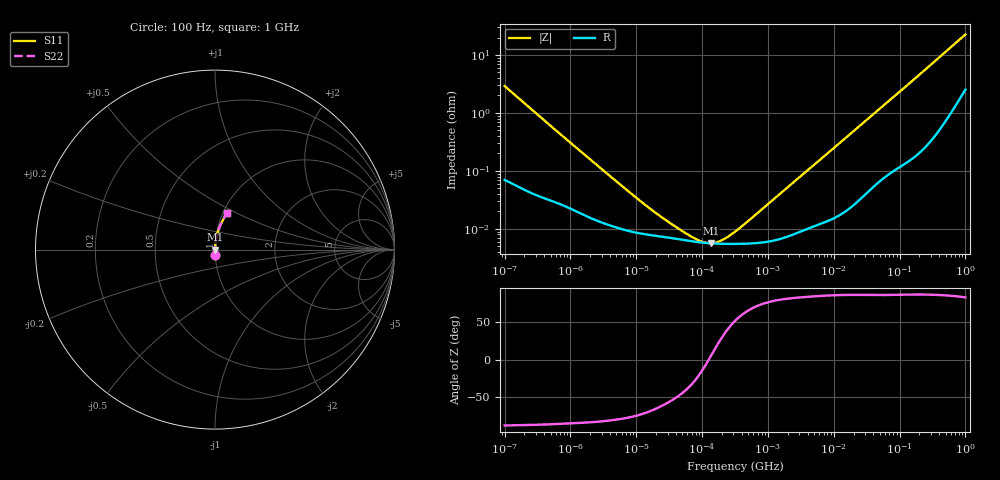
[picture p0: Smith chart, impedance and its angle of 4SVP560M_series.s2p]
!  *** S-Parameter ***
!  Copyright (C) Panasonic Industry Corporation
!  Conductive Polymer Aluminum Soild Capacitor (OS-CON)
!  Parts No. 4SVP560M
!  Connection Mode : Series
!  1  o---||---o  2
!  GND o--------o GND
!  Conditions : Temperature = 20 degC  DC Bias = 0 V
! Frequency Range : 100Hz  -  1GHz  [ 401 Steps ]
# Hz S RI R 50
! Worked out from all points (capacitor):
!   401 points, 100 Hz to 1 GHz, reference 50 ohm
!   read as one part in series: C = 545 uF near 108.4 Hz
!   lowest |Z| = 5.66 mohm at 135.7 kHz (marker M1)
!   series resonance near 126.6 kHz, so ESL is about 2.9 nH
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100  0.00154 -0.029  0.9985 0.029  0.9985 0.029  0.00154 -0.029
108.3927  0.00139 -0.0268  0.9986 0.0268  0.9986 0.0268  0.00139 -0.0268
309.0295  0.000469 -0.00957  0.9995 0.00957  0.9995 0.00957  0.000469 -0.00957
1487.647  0.000184 -0.00208  0.9998 0.00208  0.9998 0.00208  0.000184 -0.00208
9120.108  8.8e-05 -0.000365  0.9999 0.000365  0.9999 0.000365  8.8e-05 -0.000365
14791.08  7.96e-05 -0.000228  0.9999 0.000228  0.9999 0.000228  7.96e-05 -0.000228
22130.95  7.46e-05 -0.000154  0.9999 0.000154  0.9999 0.000154  7.46e-05 -0.000154
40504.19  6.73e-05 -8.32e-05  0.9999 8.32e-05  0.9999 8.32e-05  6.73e-05 -8.32e-05
45708.82  6.58e-05 -7.25e-05  0.9999 7.25e-05  0.9999 7.25e-05  6.58e-05 -7.25e-05
135675.1  5.64e-05 4.59e-06  0.9999 -4.59e-06  0.9999 -4.59e-06  5.64e-05 4.59e-06
316227.8  5.5e-05 7.04e-05  0.9999 -7.04e-05  0.9999 -7.04e-05  5.5e-05 7.04e-05
356861.7  5.51e-05 8.28e-05  0.9999 -8.28e-05  0.9999 -8.28e-05  5.51e-05 8.28e-05
402717  5.53e-05 9.64e-05  0.9999 -9.64e-05  0.9999 -9.64e-05  5.53e-05 9.64e-05
4704354  0.000109 0.00119  0.9999 -0.00119  0.9999 -0.00119  0.000109 0.00119
2.357762e7  0.000335 0.00573  0.9997 -0.00573  0.9997 -0.00573  0.000335 0.00573
6.99842e7  0.00115 0.0163  0.9988 -0.0163  0.9988 -0.0163  0.00115 0.0163
1.631173e8  0.00307 0.0371  0.9969 -0.0371  0.9969 -0.0371  0.00307 0.0371
3.108136e8  0.00836 0.0698  0.9916 -0.0698  0.9916 -0.0698  0.00836 0.0698
4.290422e8  0.0148 0.0953  0.9852 -0.0953  0.9852 -0.0953  0.0148 0.0953
5.922431e8  0.0267 0.1291  0.9733 -0.1291  0.9733 -0.1291  0.0267 0.1291
9.225714e8  0.06 0.1908  0.94 -0.1908  0.94 -0.1908  0.06 0.1908
1e9  0.0692 0.2037  0.9308 -0.2037  0.9308 -0.2037  0.0692 0.2037
